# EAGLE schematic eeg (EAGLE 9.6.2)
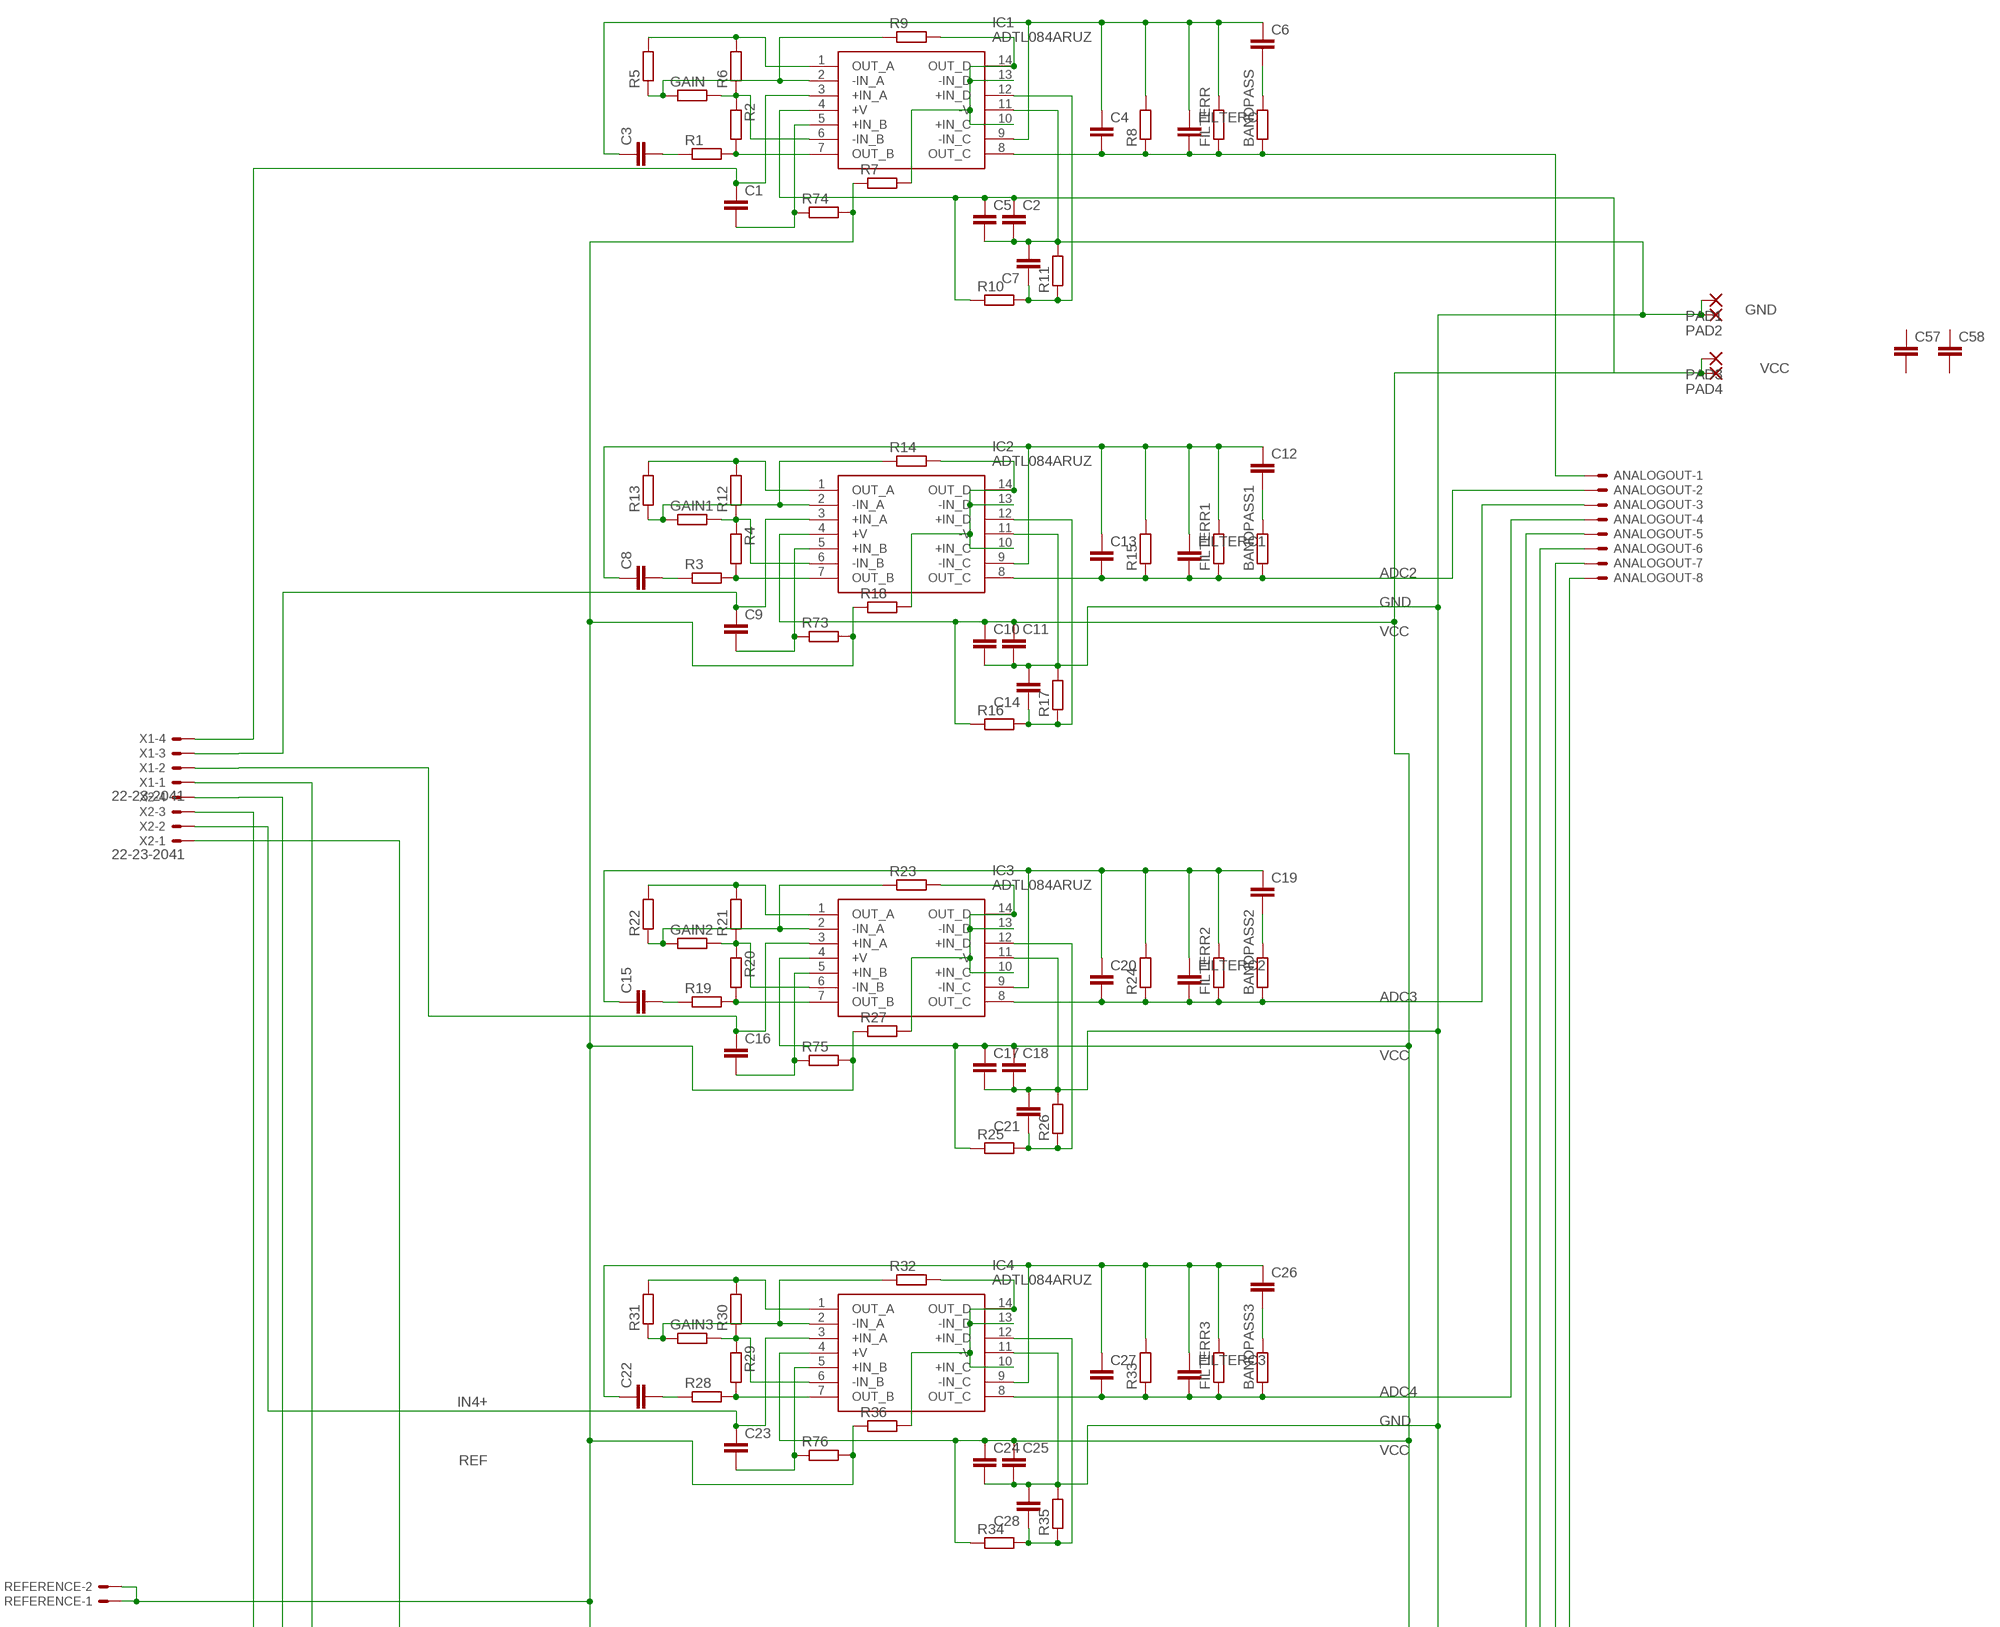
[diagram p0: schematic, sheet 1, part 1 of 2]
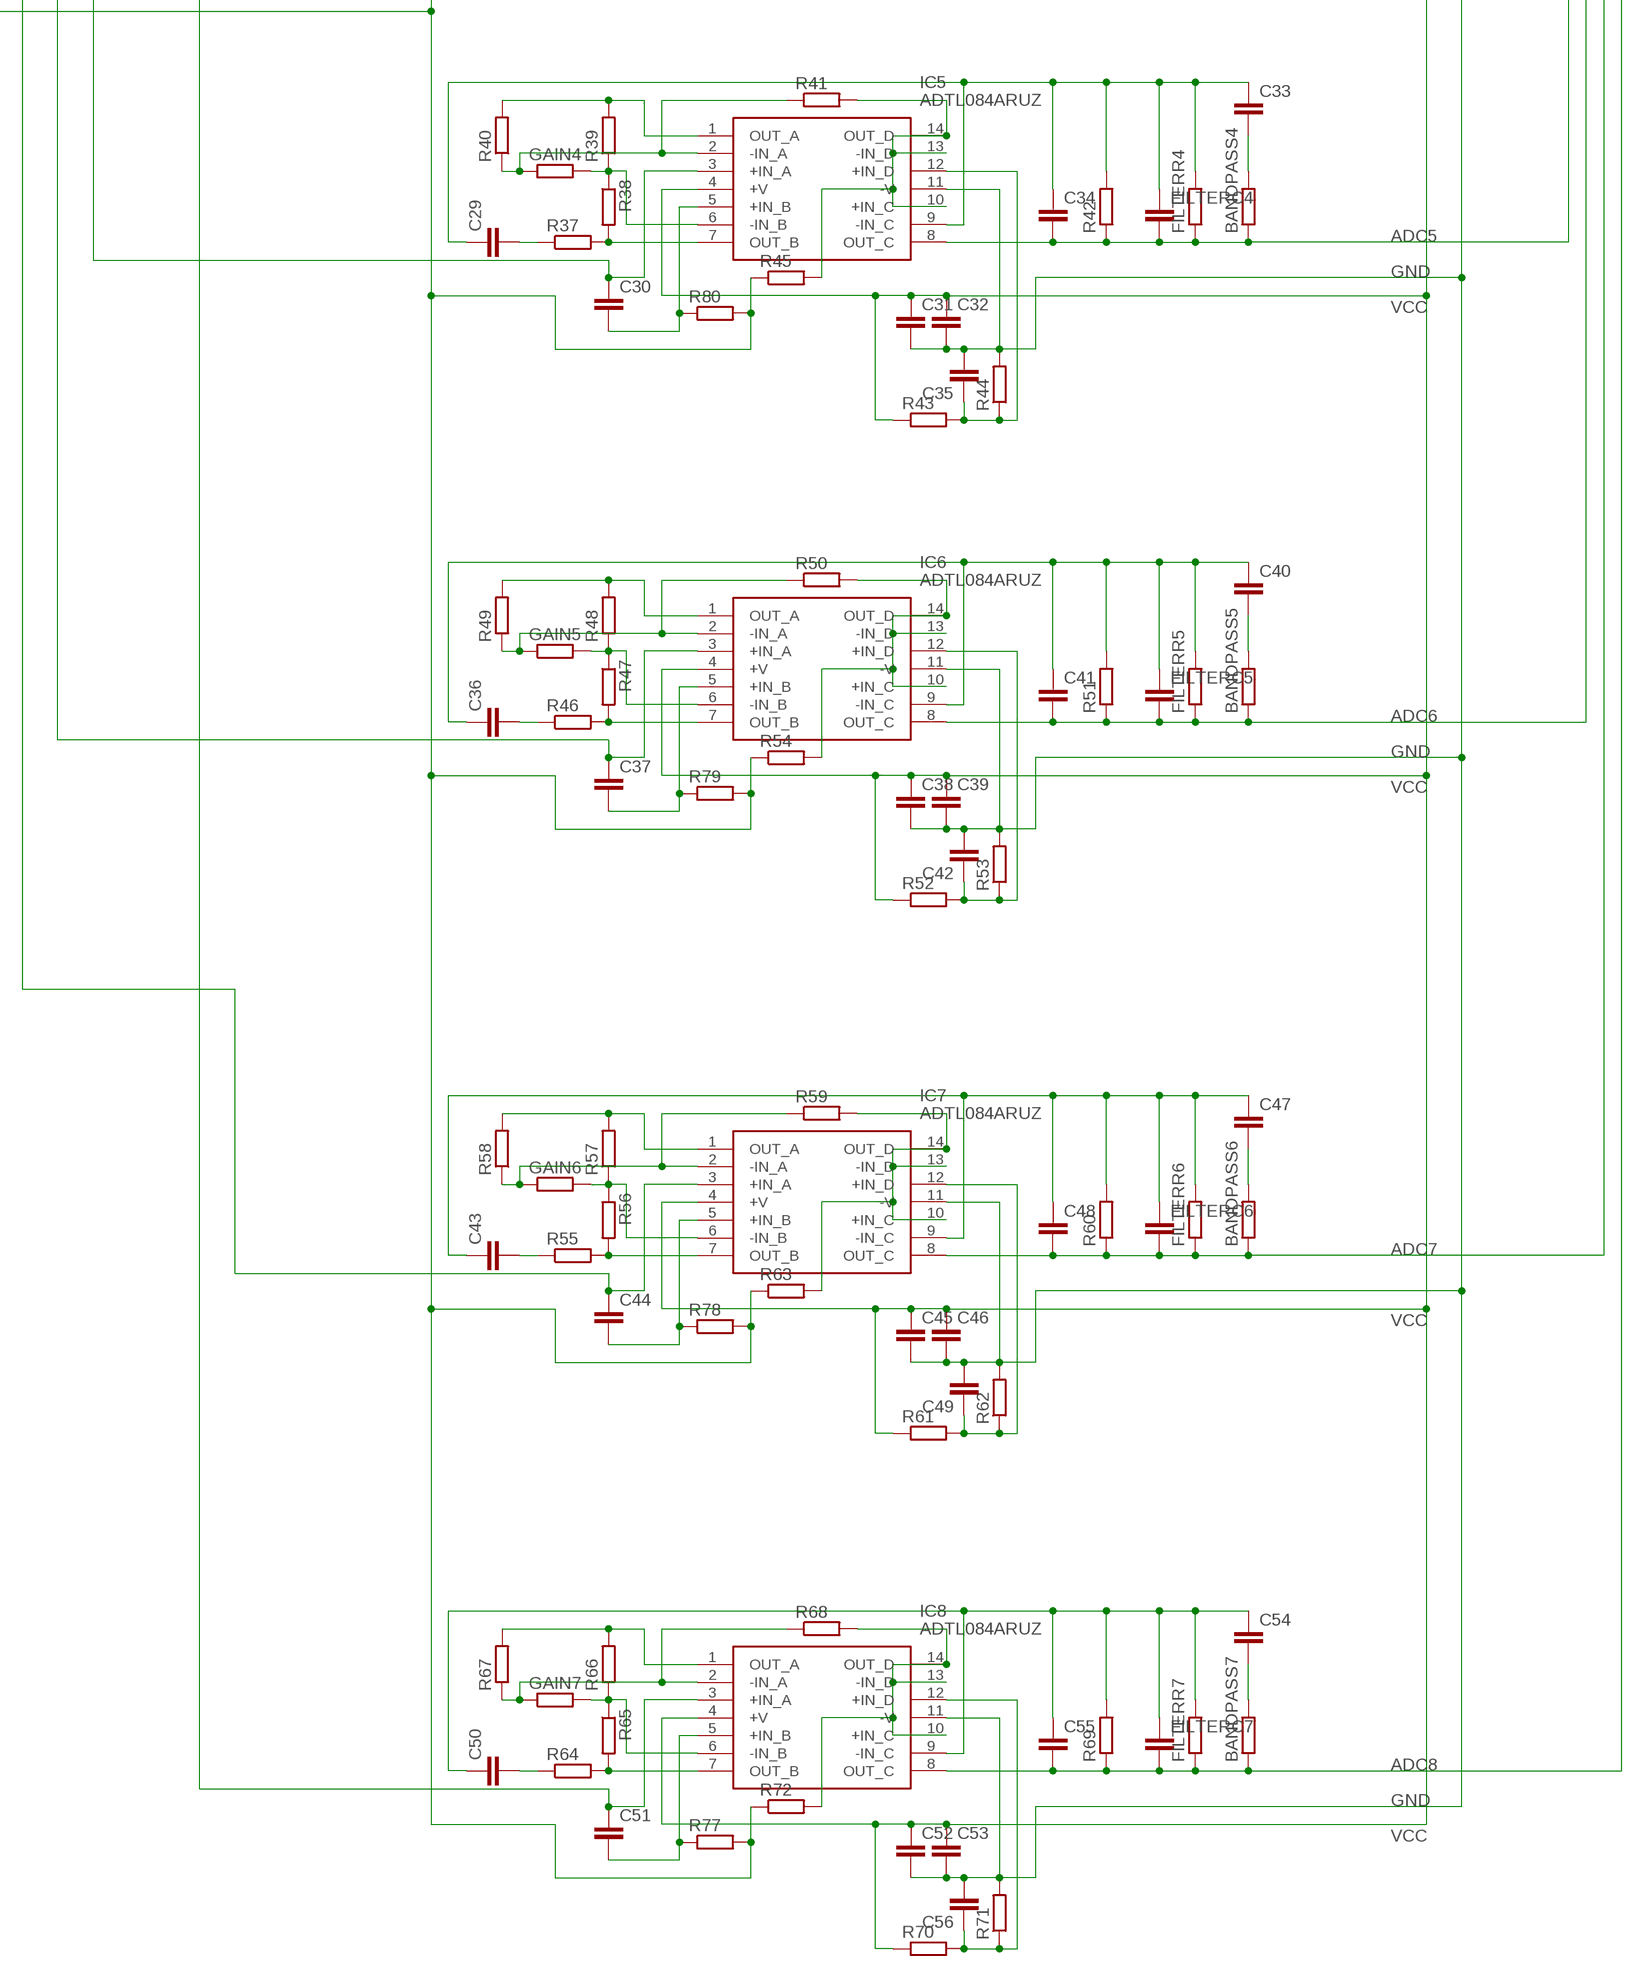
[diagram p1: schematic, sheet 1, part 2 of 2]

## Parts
ANALOGOUT  22-23-2081  [22-23-2081]
BANDPASS  R-EU_R0603  [R0603]
BANDPASS1  R-EU_R0603  [R0603]
BANDPASS2  R-EU_R0603  [R0603]
BANDPASS3  R-EU_R0603  [R0603]
BANDPASS4  R-EU_R0603  [R0603]
BANDPASS5  R-EU_R0603  [R0603]
BANDPASS6  R-EU_R0603  [R0603]
BANDPASS7  R-EU_R0603  [R0603]
C1  C-EUC0603  [C0603]
C2  C-EUC0603  [C0603]
C3  C-EUC0805  [C0805]
C4  C-EUC0603  [C0603]
C5  C-EUC0603  [C0603]
C6  C-EUC0603  [C0603]
C7  C-EUC0603  [C0603]
C8  C-EUC0805  [C0805]
C9  C-EUC0603  [C0603]
C10  C-EUC0603  [C0603]
C11  C-EUC0603  [C0603]
C12  C-EUC0603  [C0603]
C13  C-EUC0603  [C0603]
C14  C-EUC0603  [C0603]
C15  C-EUC0805  [C0805]
C16  C-EUC0603  [C0603]
C17  C-EUC0603  [C0603]
C18  C-EUC0603  [C0603]
C19  C-EUC0603  [C0603]
C20  C-EUC0603  [C0603]
C21  C-EUC0603  [C0603]
C22  C-EUC0805  [C0805]
C23  C-EUC0603  [C0603]
C24  C-EUC0603  [C0603]
C25  C-EUC0603  [C0603]
C26  C-EUC0603  [C0603]
C27  C-EUC0603  [C0603]
C28  C-EUC0603  [C0603]
C29  C-EUC0805  [C0805]
C30  C-EUC0603  [C0603]
C31  C-EUC0603  [C0603]
C32  C-EUC0603  [C0603]
C33  C-EUC0603  [C0603]
C34  C-EUC0603  [C0603]
C35  C-EUC0603  [C0603]
C36  C-EUC0805  [C0805]
C37  C-EUC0603  [C0603]
C38  C-EUC0603  [C0603]
C39  C-EUC0603  [C0603]
C40  C-EUC0603  [C0603]
C41  C-EUC0603  [C0603]
C42  C-EUC0603  [C0603]
C43  C-EUC0805  [C0805]
C44  C-EUC0603  [C0603]
C45  C-EUC0603  [C0603]
C46  C-EUC0603  [C0603]
C47  C-EUC0603  [C0603]
C48  C-EUC0603  [C0603]
C49  C-EUC0603  [C0603]
C50  C-EUC0805  [C0805]
C51  C-EUC0603  [C0603]
C52  C-EUC0603  [C0603]
C53  C-EUC0603  [C0603]
C54  C-EUC0603  [C0603]
C55  C-EUC0603  [C0603]
C56  C-EUC0603  [C0603]
C57  C-EUC0805  [C0805]
C58  C-EUC0805  [C0805]
FILTERC  C-EUC0603  [C0603]
FILTERC1  C-EUC0603  [C0603]
FILTERC2  C-EUC0603  [C0603]
FILTERC3  C-EUC0603  [C0603]
FILTERC4  C-EUC0603  [C0603]
FILTERC5  C-EUC0603  [C0603]
FILTERC6  C-EUC0603  [C0603]
FILTERC7  C-EUC0603  [C0603]
FILTERR  R-EU_R0603  [R0603]
FILTERR1  R-EU_R0603  [R0603]
FILTERR2  R-EU_R0603  [R0603]
FILTERR3  R-EU_R0603  [R0603]
FILTERR4  R-EU_R0603  [R0603]
FILTERR5  R-EU_R0603  [R0603]
FILTERR6  R-EU_R0603  [R0603]
FILTERR7  R-EU_R0603  [R0603]
GAIN  R-EU_R0603  [R0603]
GAIN1  R-EU_R0603  [R0603]
GAIN2  R-EU_R0603  [R0603]
GAIN3  R-EU_R0603  [R0603]
GAIN4  R-EU_R0603  [R0603]
GAIN5  R-EU_R0603  [R0603]
GAIN6  R-EU_R0603  [R0603]
GAIN7  R-EU_R0603  [R0603]
IC1  ADTL084ARUZ  [SOP65P640X120-14N]
IC2  ADTL084ARUZ  [SOP65P640X120-14N]
IC3  ADTL084ARUZ  [SOP65P640X120-14N]
IC4  ADTL084ARUZ  [SOP65P640X120-14N]
IC5  ADTL084ARUZ  [SOP65P640X120-14N]
IC6  ADTL084ARUZ  [SOP65P640X120-14N]
IC7  ADTL084ARUZ  [SOP65P640X120-14N]
IC8  ADTL084ARUZ  [SOP65P640X120-14N]
PAD1  2,54/1,1  [2,54/1,1]
PAD2  2,54/1,1  [2,54/1,1]
PAD3  2,54/1,1  [2,54/1,1]
PAD4  2,54/1,1  [2,54/1,1]
R1  R-EU_R0603  [R0603]
R2  R-EU_R0603  [R0603]
R3  R-EU_R0603  [R0603]
R4  R-EU_R0603  [R0603]
R5  R-EU_R0603  [R0603]
R6  R-EU_R0603  [R0603]
R7  R-EU_R0603  [R0603]
R8  R-EU_R0603  [R0603]
R9  R-EU_R0603  [R0603]
R10  R-EU_R0603  [R0603]
R11  R-EU_R0603  [R0603]
R12  R-EU_R0603  [R0603]
R13  R-EU_R0603  [R0603]
R14  R-EU_R0603  [R0603]
R15  R-EU_R0603  [R0603]
R16  R-EU_R0603  [R0603]
R17  R-EU_R0603  [R0603]
R18  R-EU_R0603  [R0603]
R19  R-EU_R0603  [R0603]
R20  R-EU_R0603  [R0603]
R21  R-EU_R0603  [R0603]
R22  R-EU_R0603  [R0603]
R23  R-EU_R0603  [R0603]
R24  R-EU_R0603  [R0603]
R25  R-EU_R0603  [R0603]
R26  R-EU_R0603  [R0603]
R27  R-EU_R0603  [R0603]
R28  R-EU_R0603  [R0603]
R29  R-EU_R0603  [R0603]
R30  R-EU_R0603  [R0603]
R31  R-EU_R0603  [R0603]
R32  R-EU_R0603  [R0603]
R33  R-EU_R0603  [R0603]
R34  R-EU_R0603  [R0603]
R35  R-EU_R0603  [R0603]
R36  R-EU_R0603  [R0603]
R37  R-EU_R0603  [R0603]
R38  R-EU_R0603  [R0603]
R39  R-EU_R0603  [R0603]
R40  R-EU_R0603  [R0603]
R41  R-EU_R0603  [R0603]
R42  R-EU_R0603  [R0603]
R43  R-EU_R0603  [R0603]
R44  R-EU_R0603  [R0603]
R45  R-EU_R0603  [R0603]
R46  R-EU_R0603  [R0603]
R47  R-EU_R0603  [R0603]
R48  R-EU_R0603  [R0603]
R49  R-EU_R0603  [R0603]
R50  R-EU_R0603  [R0603]
R51  R-EU_R0603  [R0603]
R52  R-EU_R0603  [R0603]
R53  R-EU_R0603  [R0603]
R54  R-EU_R0603  [R0603]
R55  R-EU_R0603  [R0603]
R56  R-EU_R0603  [R0603]
R57  R-EU_R0603  [R0603]
R58  R-EU_R0603  [R0603]
R59  R-EU_R0603  [R0603]
R60  R-EU_R0603  [R0603]
R61  R-EU_R0603  [R0603]
R62  R-EU_R0603  [R0603]
R63  R-EU_R0603  [R0603]
R64  R-EU_R0603  [R0603]
R65  R-EU_R0603  [R0603]
R66  R-EU_R0603  [R0603]
R67  R-EU_R0603  [R0603]
R68  R-EU_R0603  [R0603]
R69  R-EU_R0603  [R0603]
R70  R-EU_R0603  [R0603]
R71  R-EU_R0603  [R0603]
R72  R-EU_R0603  [R0603]
R73  R-EU_R0603  [R0603]
R74  R-EU_R0603  [R0603]
R75  R-EU_R0603  [R0603]
R76  R-EU_R0603  [R0603]
R77  R-EU_R0603  [R0603]
R78  R-EU_R0603  [R0603]
R79  R-EU_R0603  [R0603]
R80  R-EU_R0603  [R0603]
REFERENCE  22-23-2021  [22-23-2021]
X1  22-23-2041  [22-23-2041]
X2  22-23-2041  [22-23-2041]

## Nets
ADC1: ANALOGOUT.1 BANDPASS.1 C4.2 FILTERC.2 FILTERR.1 IC1.8(OUT_C) R8.1
ADC2: ANALOGOUT.2 BANDPASS1.1 C13.2 FILTERC1.2 FILTERR1.1 IC2.8(OUT_C) R15.1
ADC3: ANALOGOUT.3 BANDPASS2.1 C20.2 FILTERC2.2 FILTERR2.1 IC3.8(OUT_C) R24.1
ADC4: ANALOGOUT.4 BANDPASS3.1 C27.2 FILTERC3.2 FILTERR3.1 IC4.8(OUT_C) R33.1
ADC5: ANALOGOUT.5 BANDPASS4.1 C34.2 FILTERC4.2 FILTERR4.1 IC5.8(OUT_C) R42.1
ADC6: ANALOGOUT.6 BANDPASS5.1 C41.2 FILTERC5.2 FILTERR5.1 IC6.8(OUT_C) R51.1
ADC7: ANALOGOUT.7 BANDPASS6.1 C48.2 FILTERC6.2 FILTERR6.1 IC7.8(OUT_C) R60.1
ADC8: ANALOGOUT.8 BANDPASS7.1 C55.2 FILTERC7.2 FILTERR7.1 IC8.8(OUT_C) R69.1
B$1: C3.1 C4.1 C6.1 FILTERC.1 FILTERR.2 IC1.9(-IN_C) R8.2
B$2: C8.1 C12.1 C13.1 FILTERC1.1 FILTERR1.2 IC2.9(-IN_C) R15.2
B$3: C15.1 C19.1 C20.1 FILTERC2.1 FILTERR2.2 IC3.9(-IN_C) R24.2
B$4: C22.1 C26.1 C27.1 FILTERC3.1 FILTERR3.2 IC4.9(-IN_C) R33.2
B$5: C29.1 C33.1 C34.1 FILTERC4.1 FILTERR4.2 IC5.9(-IN_C) R42.2
B$6: C36.1 C40.1 C41.1 FILTERC5.1 FILTERR5.2 IC6.9(-IN_C) R51.2
B$7: C43.1 C47.1 C48.1 FILTERC6.1 FILTERR6.2 IC7.9(-IN_C) R60.2
B$8: C50.1 C54.1 C55.1 FILTERC7.1 FILTERR7.2 IC8.9(-IN_C) R69.2
GND: C2.2 C5.2 C7.2 C10.2 C11.2 C14.2 C17.2 C18.2 C21.2 C24.2 C25.2 C28.2 C31.2 C32.2 C35.2 C38.2 C39.2 C42.2 C45.2 C46.2 C49.2 C52.2 C53.2 C56.2 IC1.11(-V) IC2.11(-V) IC3.11(-V) IC4.11(-V) IC5.11(-V) IC6.11(-V) IC7.11(-V) IC8.11(-V) PAD1.1(P) PAD2.1(P) R11.2 R17.2 R26.2 R35.2 R44.2 R53.2 R62.2 R71.2
IN1+: C1.1 IC1.3(+IN_A) X1.4
IN2+: C9.1 IC2.3(+IN_A) X1.3
IN2-: C9.2 IC2.5(+IN_B) R73.1
IN3+: C16.1 IC3.3(+IN_A) X1.2
IN4+: C23.1 IC4.3(+IN_A) X2.2
IN5+: C30.1 IC5.3(+IN_A) X1.1
IN6+: C37.1 IC6.3(+IN_A) X2.4
IN7+: C44.1 IC7.3(+IN_A) X2.3
IN8+: C51.1 IC8.3(+IN_A) X2.1
N$1: IC1.7(OUT_B) R1.2 R2.2
N$2: C3.2 R1.1
N$3: GAIN.2 IC1.6(-IN_B) R2.1 R6.1
N$4: IC1.1(OUT_A) R5.2 R6.2
N$5: IC2.7(OUT_B) R3.2 R4.2
N$6: IC1.10(+IN_C) IC1.13(-IN_D) IC1.14(OUT_D) R7.2 R9.2
N$7: GAIN.1 IC1.2(-IN_A) R5.1 R9.1
N$8: GAIN1.2 IC2.6(-IN_B) R4.1 R12.1
N$9: IC2.1(OUT_A) R12.2 R13.2
N$10: IC2.10(+IN_C) IC2.13(-IN_D) IC2.14(OUT_D) R14.2 R18.2
N$11: BANDPASS.2 C6.2
N$12: C7.1 IC1.12(+IN_D) R10.2 R11.1
N$13: GAIN1.1 IC2.2(-IN_A) R13.1 R14.1
N$14: C8.2 R3.1
N$15: BANDPASS1.2 C12.2
N$16: C14.1 IC2.12(+IN_D) R16.2 R17.1
N$17: IC3.7(OUT_B) R19.2 R20.2
N$18: GAIN2.2 IC3.6(-IN_B) R20.1 R21.1
N$19: IC3.1(OUT_A) R21.2 R22.2
N$20: IC3.10(+IN_C) IC3.13(-IN_D) IC3.14(OUT_D) R23.2 R27.2
N$21: GAIN2.1 IC3.2(-IN_A) R22.1 R23.1
N$22: C15.2 R19.1
N$23: BANDPASS2.2 C19.2
N$24: C21.1 IC3.12(+IN_D) R25.2 R26.1
N$25: IC4.7(OUT_B) R28.2 R29.2
N$26: GAIN3.2 IC4.6(-IN_B) R29.1 R30.1
N$27: IC4.1(OUT_A) R30.2 R31.2
N$28: IC4.10(+IN_C) IC4.13(-IN_D) IC4.14(OUT_D) R32.2 R36.2
N$29: GAIN3.1 IC4.2(-IN_A) R31.1 R32.1
N$30: C22.2 R28.1
N$31: BANDPASS3.2 C26.2
N$32: C28.1 IC4.12(+IN_D) R34.2 R35.1
N$33: IC5.7(OUT_B) R37.2 R38.2
N$34: GAIN4.2 IC5.6(-IN_B) R38.1 R39.1
N$35: IC5.1(OUT_A) R39.2 R40.2
N$36: IC5.10(+IN_C) IC5.13(-IN_D) IC5.14(OUT_D) R41.2 R45.2
N$37: GAIN4.1 IC5.2(-IN_A) R40.1 R41.1
N$38: C29.2 R37.1
N$39: BANDPASS4.2 C33.2
N$40: C35.1 IC5.12(+IN_D) R43.2 R44.1
N$41: IC6.7(OUT_B) R46.2 R47.2
N$42: GAIN5.2 IC6.6(-IN_B) R47.1 R48.1
N$43: IC6.1(OUT_A) R48.2 R49.2
N$44: IC6.10(+IN_C) IC6.13(-IN_D) IC6.14(OUT_D) R50.2 R54.2
N$45: GAIN5.1 IC6.2(-IN_A) R49.1 R50.1
N$46: C36.2 R46.1
N$47: BANDPASS5.2 C40.2
N$48: C42.1 IC6.12(+IN_D) R52.2 R53.1
N$49: IC7.7(OUT_B) R55.2 R56.2
N$50: GAIN6.2 IC7.6(-IN_B) R56.1 R57.1
N$51: IC7.1(OUT_A) R57.2 R58.2
N$52: IC7.10(+IN_C) IC7.13(-IN_D) IC7.14(OUT_D) R59.2 R63.2
N$53: GAIN6.1 IC7.2(-IN_A) R58.1 R59.1
N$54: C43.2 R55.1
N$55: BANDPASS6.2 C47.2
N$56: C49.1 IC7.12(+IN_D) R61.2 R62.1
N$57: IC8.7(OUT_B) R64.2 R65.2
N$58: GAIN7.2 IC8.6(-IN_B) R65.1 R66.1
N$59: IC8.1(OUT_A) R66.2 R67.2
N$60: IC8.10(+IN_C) IC8.13(-IN_D) IC8.14(OUT_D) R68.2 R72.2
N$61: GAIN7.1 IC8.2(-IN_A) R67.1 R68.1
N$62: C50.2 R64.1
N$63: BANDPASS7.2 C54.2
N$64: C56.1 IC8.12(+IN_D) R70.2 R71.1
N$65: C1.2 IC1.5(+IN_B) R74.1
N$67: C51.2 IC8.5(+IN_B) R77.1
N$68: C44.2 IC7.5(+IN_B) R78.1
N$69: C37.2 IC6.5(+IN_B) R79.1
N$70: C30.2 IC5.5(+IN_B) R80.1
N$71: C23.2 IC4.5(+IN_B) R76.1
N$72: C16.2 IC3.5(+IN_B) R75.1
REF: R7.1 R18.1 R27.1 R36.1 R45.1 R54.1 R63.1 R72.1 R73.2 R74.2 R75.2 R76.2 R77.2 R78.2 R79.2 R80.2 REFERENCE.1 REFERENCE.2
VCC: C2.1 C5.1 C10.1 C11.1 C17.1 C18.1 C24.1 C25.1 C31.1 C32.1 C38.1 C39.1 C45.1 C46.1 C52.1 C53.1 IC1.4(+V) IC2.4(+V) IC3.4(+V) IC4.4(+V) IC5.4(+V) IC6.4(+V) IC7.4(+V) IC8.4(+V) PAD3.1(P) PAD4.1(P) R10.1 R16.1 R25.1 R34.1 R43.1 R52.1 R61.1 R70.1
Unconnected: C57.1 C57.2 C58.1 C58.2

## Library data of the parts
ANALOGOUT = con-molex:22-23-2081: .100" (2.54mm) Center Header - 8 Pin; MF: MOLEX; MPN: 22-23-2081; OC_FARNELL: 1756826; OC_NEWARK: 01C7592
BANDPASS BANDPASS1-BANDPASS7 FILTERR FILTERR1-FILTERR7 GAIN GAIN1-GAIN7 R1-R80 = rcl:R-EU_: RESISTOR, European symbol; SPICEPREFIX: R
C1-C58 FILTERC FILTERC1-FILTERC7 = rcl:C-EU: CAPACITOR, European symbol; SPICEPREFIX: C
IC1-IC8 = ADTL084ARUZ:ADTL084ARUZ: ADTL084ARUZ, Quad Operational Amplifier 5MHz, 14-Pin TSSOP Source: Datasheet; ARROW_PART_NUMBER: ADTL084ARUZ; ARROW_PRICE-STOCK: https://www.arrow.com/en/products/adtl084aruz/analog-devices; DESCRIPTION: ADTL084ARUZ, Quad Operational Amplifier 5MHz, 14-Pin TSSOP; HEIGHT: 1.2mm; MANUFACTURER_NAME: Analog Devices; MANUFACTURER_PART_NUMBER: ADTL084ARUZ; MOUSER_PART_NUMBER: 584-ADTL084ARUZ; MOUSER_PRICE-STOCK: https://www.mouser.co.uk/ProductDetail/Analog-Devices/ADTL084ARUZ?qs=WIvQP4zGanh2v1vzKZRzoA%3D%3D
PAD1-PAD4 = wirepad:2,54/1,1: THROUGH-HOLE PAD
REFERENCE = con-molex:22-23-2021: .100" (2.54mm) Center Header - 2 Pin; MF: MOLEX; MPN: 22-23-2021; OC_FARNELL: 1462926; OC_NEWARK: 25C3832
X1 X2 = con-molex:22-23-2041: .100" (2.54mm) Center Header - 4 Pin; MF: MOLEX; MPN: 22-23-2041; OC_FARNELL: 1462920; OC_NEWARK: 38C0355

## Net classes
0 default: clearance 0.205 mm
